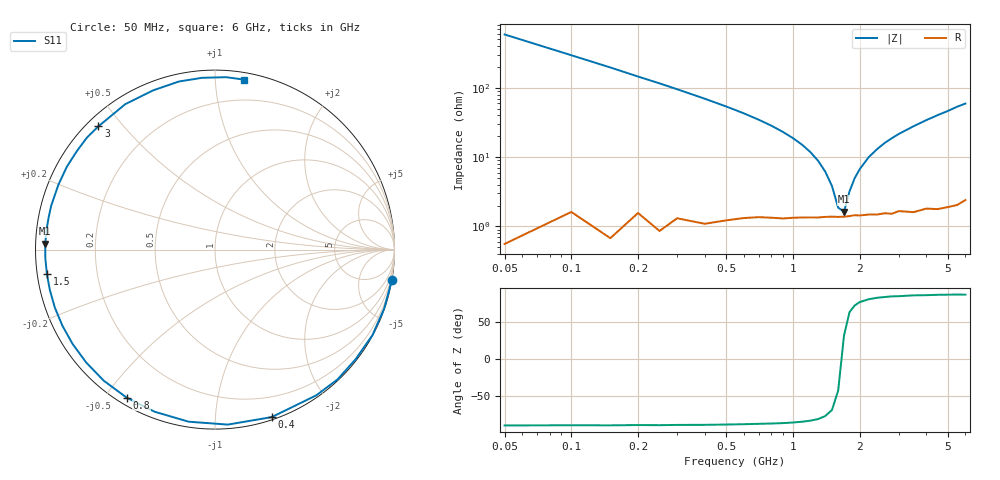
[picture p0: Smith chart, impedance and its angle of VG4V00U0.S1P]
! Infineon Technologies  Discrete & RF Semiconductors
! BB 831
! Si Tuning Diode in SOD323
! VR = 4 V
! S-Parameters:  July  1999
# GHz  S  MA  R  50
!  f  S11
! GHz  MAG  ANG
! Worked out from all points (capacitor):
!   34 points, 50 MHz to 6 GHz, reference 50 ohm
!   read as one part to ground: C = 5.36 pF near 50 MHz
!   lowest |Z| = 1.64 ohm at 1.7 GHz (marker M1)
!   series resonance near 1.659 GHz, so ESL is about 1.7 nH
!   S11 on the Smith chart (normalised r, x): 50 MHz: 0, -12; 400 MHz: 0.02, -1.39; 800 MHz: 0.03, -0.57; 1.5 GHz: 0.03, -0.07; 3 GHz: 0.03, +0.43; 6 GHz: 0.05, +1.19
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0.05  0.9998 -9.7
0.1  0.9982 -19.2
0.15  0.9984 -28.5
0.2  0.9934 -37.9
0.25  0.9946 -46.6
0.3  0.9888 -55.2
0.4  0.9853 -71.3
0.5  0.9776 -85.8
0.6  0.97 -98.7
0.7  0.9639 -110.4
0.8  0.9604 -120.8
0.9  0.9579 -130.3
1  0.9543 -138.8
1.1  0.9518 -146.5
1.3  0.949 -160.2
1.5  0.9464 -171.8
1.6  0.9466 -177.1
1.7  0.9462 178.0
2  0.9449 165.1
2.4  0.9458 150.8
2.6  0.9453 144.4
3  0.9453 133.4
3.5  0.9521 121.7
4  0.9518 111.2
4.5  0.9579 102.1
5  0.9599 94.3
5.5  0.9626 86.3
6  0.9608 80.2
